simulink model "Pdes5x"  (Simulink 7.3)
settings: Solver=ode45  StartTime=0.0  StopTime=50  RelTol=1e-3
undefined symbols (not defined in the file or in its folder): Aps, Bps, Cps, Dps, Kmix

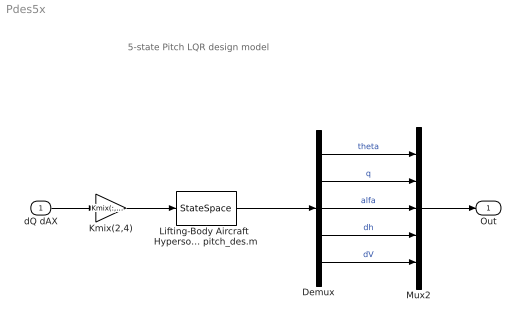
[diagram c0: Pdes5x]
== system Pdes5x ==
  note: 5-state Pitch LQR design model
  dQ dAX : Inport  OutDataType=sfix(16)  OutScaling=2^0
  Demux : Demux  Outputs=5
  Kmix(2,4) : Gain  Gain=Kmix(:, [2,4])  Multiplication=Matrix(K*u)  ParameterDataType=sfix(16)  ParameterScaling=2^0  OutDataType=sfix(16)  OutScaling=2^0
  Lifting-Body Aircraft  Hypersonic Pitch  Design Model from file pitch_des.m : StateSpace  A=Aps  B=Bps  C=Cps  D=Dps
  Mux2 : Mux  Inputs=5
  Out : Outport  OutDataType=sfix(16)  OutScaling=2^0
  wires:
  Lifting-Body Aircraft  Hypersonic Pitch  Design Model from file pitch_des.m/1 -> Demux/1
  dQ dAX/1 -> Kmix(2,4)/1
  Mux2/1 -> Out/1
  Demux/1 -> Mux2/1  "theta"
  Demux/2 -> Mux2/2  "q"
  Demux/3 -> Mux2/3  "alfa"
  Demux/4 -> Mux2/4  "dh"
  Demux/5 -> Mux2/5  "dV"
  Kmix(2,4)/1 -> Lifting-Body Aircraft  Hypersonic Pitch  Design Model from file pitch_des.m/1
